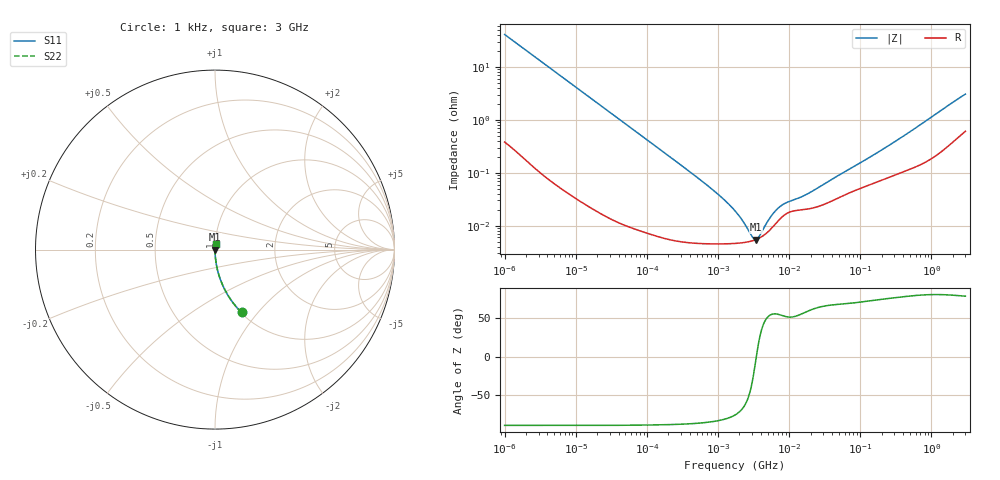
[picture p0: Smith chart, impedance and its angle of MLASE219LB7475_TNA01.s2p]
! MLASE219LB7475_TNA01  S-PARAMETER MODEL  ( Standard Model )
! Model Generated by TAIYO YUDEN Corporation (http://www.ty-top.com)
! Version 1.0
! TAIYO YUDEN Control No. 220601
! Copyright(c) 2014 TAIYO YUDEN CO.,LTD. All Rights Reserved.
! Product Description (link to TY-COMPAS)
! https://ds.yuden.co.jp/TYCOMPAS/or/detail?pn=MLASE219LB7475MTNA01&u=M
! Products Name : Multilayer Ceramic Capacitors
! Characteristics :
!  Capacitance : 4.7 [uF] , Rated Voltage : 16 [V] , TCC : X7R
!  Case Size : 2.0 x 1.25 / 0.079 x 0.049 [mm/inch] , Thickness : 0.85 / 0.033 [mm/inch]
!  (Conditions: Temperature = 25 [degC] , DC Bias Voltage = 0 [V])
! External Node Assignments :
!  1  o---| |---o  2
! GND o---------o GND
! Frequency Range : 1kHz  -  3GHz  [ 401 STEP ]
# MHZ S RI R 50
! Freq[MHz].  S11 Real  S11 Imag  S21 Real  S21 Imag  S12 Real  S12 Imag  S22 Real  S22 Imag
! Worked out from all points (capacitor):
!   401 points, 1 kHz to 3 GHz, reference 50 ohm
!   read as one part in series: C = 3.85 uF near 1.077 kHz
!   lowest |Z| = 5.45 mohm at 3.389 MHz (marker M1)
!   series resonance near 3.458 MHz, so ESL is about 550 pH
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0.001  0.1479 -0.3504  0.8521 0.3504  0.8521 0.3504  0.1479 -0.3504
0.001685  0.0588 -0.2309  0.9412 0.2309  0.9412 0.2309  0.0588 -0.2309
0.003177  0.0178 -0.1284  0.9822 0.1284  0.9822 0.1284  0.0178 -0.1284
0.005768  0.00572 -0.0718  0.9943 0.0718  0.9943 0.0718  0.00572 -0.0718
0.01216  0.00145 -0.0343  0.9985 0.0343  0.9985 0.0343  0.00145 -0.0343
0.147855  6.94e-05 -0.00285  0.9999 0.00285  0.9999 0.00285  6.94e-05 -0.00285
0.791611  4.55e-05 -0.000509  1 0.000509  1 0.000509  4.55e-05 -0.000509
1.238299  4.53e-05 -0.0003  1 0.0003  1 0.0003  4.53e-05 -0.0003
1.732051  4.61e-05 -0.000185  1 0.000185  1 0.000185  4.61e-05 -0.000185
2.334012  4.8e-05 -0.000101  1 0.000101  1 0.000101  4.8e-05 -0.000101
2.514714  4.88e-05 -8.09e-05  1 8.09e-05  1 8.09e-05  4.88e-05 -8.09e-05
3.388684  5.43e-05 -5.05e-06  0.9999 5.05e-06  0.9999 5.05e-06  5.43e-05 -5.05e-06
4.399271  6.57e-05 6.16e-05  0.9999 -6.16e-05  0.9999 -6.16e-05  6.57e-05 6.16e-05
4.739869  7.1e-05 8.1e-05  0.9999 -8.1e-05  0.9999 -8.1e-05  7.1e-05 8.1e-05
6.387174  0.000107 0.000156  0.9999 -0.000156  0.9999 -0.000156  0.000107 0.000156
7.696136  0.00014 0.000192  0.9999 -0.000192  0.9999 -0.000192  0.00014 0.000192
9.273352  0.00017 0.000216  0.9998 -0.000216  0.9998 -0.000216  0.00017 0.000216
15.05716  0.000199 0.000291  0.9998 -0.000291  0.9998 -0.000291  0.000199 0.000291
21.06097  0.000214 0.000392  0.9998 -0.000392  0.9998 -0.000392  0.000214 0.000392
256.0921  0.000831 0.00323  0.9992 -0.00323  0.9992 -0.00323  0.000831 0.00323
2066.299  0.00441 0.0216  0.9956 -0.0216  0.9956 -0.0216  0.00441 0.0216
3000  0.00695 0.0298  0.9931 -0.0298  0.9931 -0.0298  0.00695 0.0298
